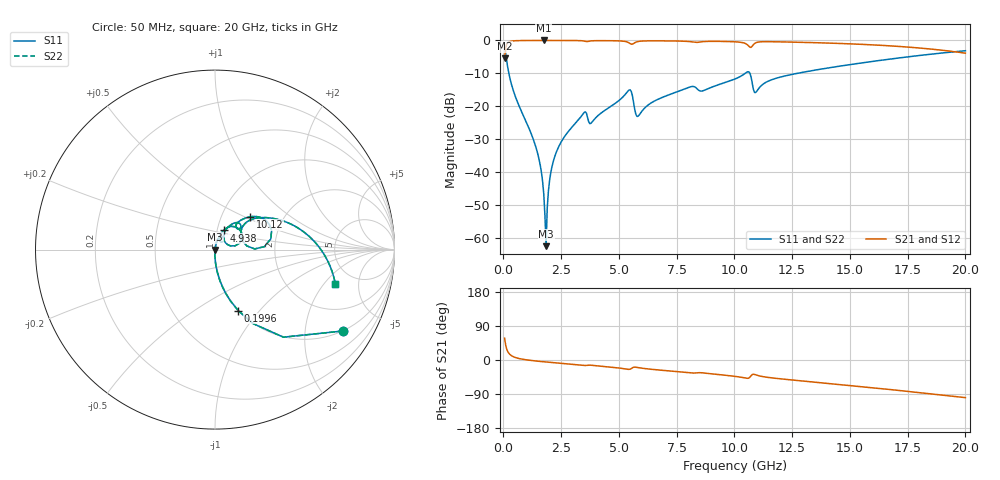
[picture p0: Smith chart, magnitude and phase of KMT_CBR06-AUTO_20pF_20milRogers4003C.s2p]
! Data measured by Modelithics Inc. support@modelithics.com 813-866-6335
! KEMET CBR06-AUTO 20pF, Pad Width= 0.851mm, Pad Length= 0.64mm, Pad Gap= 0.62mm, 20mil Rogers 4003C substrate Data, January 2022
# hz S ma R 50
! 2 Port Network Data from SP1.SP block
! freq  magS11  angS11  magS21  angS21  magS12  angS12  magS22  angS22
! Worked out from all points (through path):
!   401 points, 50 MHz to 20 GHz, reference 50 ohm
!   highest |S21| = -0.01 dB at 1.746 GHz (marker M1); lowest = -5.4 dB at 50 MHz (marker M2)
!   group delay of S21, straight-line fit = 14.2 ps
!   lowest |S11| = -62.6 dB at 1.845 GHz (marker M3), VSWR 1.00, Z = 50.1 + j0.0281 ohm
!   |S11| at or under -10 dB: 234.1 MHz to 10.47 GHz (10.23 GHz wide, 191 % of centre); 10.67 GHz to 12.73 GHz (2.053 GHz wide, 17.5 % of centre)
!   |S22| runs from -62.6 to -1.5 dB; largest |S21 - S12| = 0
!   S11 on the Smith chart (normalised r, x): 50 MHz: 0.99, -3.15; 199.6 MHz: 0.99, -0.78; 4.938 GHz: 1.07, +0.23; 10.12 GHz: 1.37, +0.54; 20 GHz: 3.53, -2.64
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5e7  0.8447 -32.5  0.5349 57.5  0.5349 57.5  0.8447 -32.5
1.99625e8  0.3643 -69.1  0.9309 20.8  0.9309 20.8  0.3643 -69.1
5.4875e8  0.1303 -83.9  0.9911 5.9  0.9911 5.9  0.1303 -83.9
1.4465e9  0.02116 -91.3  0.9991 -2.9  0.9991 -2.9  0.02116 -91.3
1.646e9  0.009753 -90.5  0.9993 -4.1  0.9993 -4.1  0.009753 -90.5
1.74575e9  0.004604 -86.7  0.9993 -4.7  0.9993 -4.7  0.004604 -86.7
1.8455e9  0.0007422 22.2  0.9993 -5.3  0.9993 -5.3  0.0007422 22.2
2.094875e9  0.01173 79.9  0.9991 -6.6  0.9991 -6.6  0.01173 79.9
2.294375e9  0.0202 80.1  0.9989 -7.7  0.9989 -7.7  0.0202 80.1
3.391625e9  0.07197 70.1  0.9896 -13.7  0.9896 -13.7  0.07197 70.1
3.790625e9  0.05496 61.0  0.984 -13.8  0.984 -13.8  0.05496 61.0
4.93775e9  0.117 66.1  0.9864 -20.7  0.9864 -20.7  0.117 66.1
5.486375e9  0.1769 34.0  0.8952 -24.2  0.8952 -24.2  0.1769 34.0
5.8355e9  0.07063 42.3  0.9651 -20.1  0.9651 -20.1  0.07063 42.3
6.73325e9  0.1293 61.1  0.9857 -26.4  0.9857 -26.4  0.1293 61.1
1.0025e10  0.2593 44.1  0.9533 -43.2  0.9533 -43.2  0.2593 44.1
1.012475e10  0.2685 42.9  0.9484 -44.0  0.9484 -44.0  0.2685 42.9
1.06235e10  0.3333 18.8  0.8182 -47.6  0.8182 -47.6  0.3333 18.8
1.092275e10  0.1617 26.0  0.9207 -39.1  0.9207 -39.1  0.1617 26.0
1.336662e10  0.3477 30.6  0.9272 -57.7  0.9272 -57.7  0.3477 30.6
1.670825e10  0.5189 9.4  0.8286 -77.7  0.8286 -77.7  0.5189 9.4
2e10  0.6972 -16.0  0.6398 -99.3  0.6398 -99.3  0.6972 -16.0
